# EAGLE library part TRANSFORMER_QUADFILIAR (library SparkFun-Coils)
Transformer with 4 independent windings
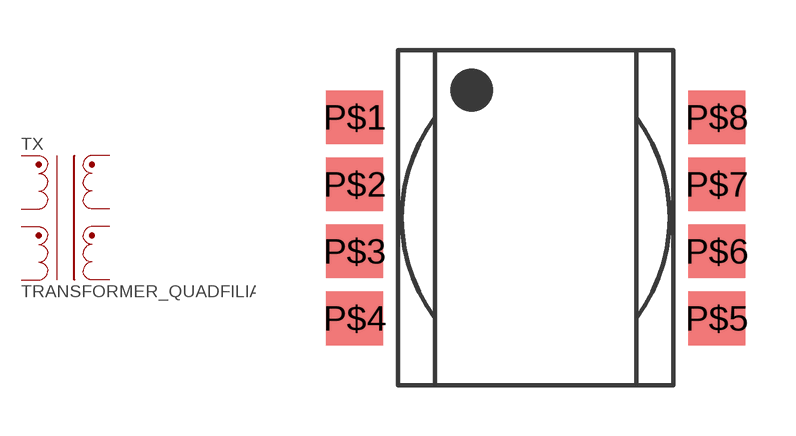
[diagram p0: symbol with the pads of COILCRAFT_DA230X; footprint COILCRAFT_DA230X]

Designator prefix TX

## TRANSFORMER_QUADFILIAR  [COILCRAFT_DA230X]
P$1  1  pas
P$2  2  pas
P$3  3  pas
P$4  4  pas
P$5  5  pas
P$6  6  pas
P$7  7  pas
P$8  8  pas

## Footprint COILCRAFT_DA230X (pad centres in mm)
Coilcraft DA2303, DA2304
smd 1.7 x 1.6: P$1 -5.4,3; P$2 -5.4,1; P$3 -5.4,-1; P$4 -5.4,-3; P$5 5.4,-3; P$6 5.4,-1; P$7 5.4,1; P$8 5.4,3

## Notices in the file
Licensing: Creative Commons ShareAlike 4.0 International - https://creativecommons.org/licenses/by-sa/4.0
